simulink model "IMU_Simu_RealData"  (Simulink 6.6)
settings: Solver=ode45  StartTime=0.0  StopTime=33.332  RelTol=1e-3
undefined symbols (not defined in the file or in its folder): float, gaind, polesd, tustin, zerosd

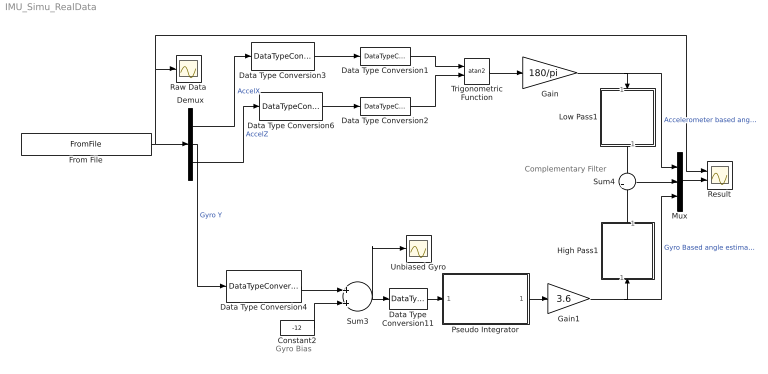
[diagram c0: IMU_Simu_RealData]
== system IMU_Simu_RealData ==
  note: Gyro Bias
  note: Complementary Filter
  Constant2 : Constant  Value=-12  SampleTime=-1
  Data Type Conversion1 : DataTypeConversion  OutDataTypeMode=single  OutScaling="[ (80/(2048*2^4))  0]"
  Data Type Conversion11 : DataTypeConversion  OutDataTypeMode=double  OutScaling="[ (80/(2048*2^4))  0]"
  Data Type Conversion2 : DataTypeConversion  OutDataTypeMode=single  OutScaling="[ (80/(2048*2^4))  0]"
  Data Type Conversion3 : DataTypeConversion  OutDataTypeMode=Specify via dialog  OutDataType=sfix(12)  OutScaling=[1/502.5*1000 0]  ConvertRealWorld=Stored Integer (SI)
  Data Type Conversion4 : DataTypeConversion  OutDataTypeMode=Specify via dialog  OutDataType=sfix(12)  OutScaling="[ (160/4096)  0]"  ConvertRealWorld=Stored Integer (SI)
  Data Type Conversion6 : DataTypeConversion  OutDataTypeMode=Specify via dialog  OutDataType=sfix(12)  OutScaling=[1/486*1000 0]  ConvertRealWorld=Stored Integer (SI)
  Demux : Demux  Outputs=3
  From File : FromFile  FileName=AxelX_GyroY_AxelZ3.mat  SampleTime=.001
  Gain : Gain  Gain=180/pi  OutDataTypeMode=Specify via dialog  OutDataType=float('double')
  Gain1 : Gain  Gain=3.6  OutDataTypeMode=Specify via dialog  OutDataType=float('double')
  High Pass1 : Subsystem  Orientation=up  mask(DiscretizedZeroPole){Zeros=[0], Poles=[-.5], Gain=1, AbsTol=auto, SampleTime=.001, method=tustin, Wc=1}
      mask prompts: Zeros "Zeros (enter in s-main:)"; Poles "Poles (enter in s-domain:)"; Gain "Gain (enter in s-domain:)"; AbsTol "Absolute tolerance:"; SampleTime "Sample time:"; Wc "Critical Frequency (Hz):"
      mask help: Continuous mask uses c2d to transform parameters onto the Discrete Zero-Pole block inside.
      mask init:
      | st=SampleTime;
      | if length(st)>1
      |     st=SampleTime(1);
      | end
      | if(st>0)
      |     [zerosd,polesd,gaind] = sldiscutil('disczpk', {st,method,Wc,Zeros,Poles,Gain});
      | end	
      | s = get_param(gcb,'maskvalues');
      | zeross = s{1};
      | poless = s{2};
      | gainss = s{3};
      | %zerosc = eval(zeross);
      | %polesc = eval(poless);
      | %gainsc = eval(gainss);
      | sldiscutil('initzpkmask', st);
      | if(st==0)
      | set_param([gcb '/Zero Pole'], 'AbsoluteTolerance', AbsTol);
      | end
  Low Pass1 : Subsystem  Orientation=down  mask(DiscretizedZeroPole){Zeros=[], Poles=[-.5], Gain=.5, AbsTol=auto, SampleTime=.001, method=tustin, Wc=1}
      mask prompts: Zeros "Zeros (enter in s-main:)"; Poles "Poles (enter in s-domain:)"; Gain "Gain (enter in s-domain:)"; AbsTol "Absolute tolerance:"; SampleTime "Sample time:"; Wc "Critical Frequency (Hz):"
      mask help: Continuous mask uses c2d to transform parameters onto the Discrete Zero-Pole block inside.
      mask init:
      | st=SampleTime;
      | if length(st)>1
      |     st=SampleTime(1);
      | end
      | if(st>0)
      |     [zerosd,polesd,gaind] = sldiscutil('disczpk', {st,method,Wc,Zeros,Poles,Gain});
      | end	
      | s = get_param(gcb,'maskvalues');
      | zeross = s{1};
      | poless = s{2};
      | gainss = s{3};
      | %zerosc = eval(zeross);
      | %polesc = eval(poless);
      | %gainsc = eval(gainss);
      | sldiscutil('initzpkmask', st);
      | if(st==0)
      | set_param([gcb '/Zero Pole'], 'AbsoluteTolerance', AbsTol);
      | end
  Mux : Mux  Inputs=3
  Pseudo Integrator : Subsystem  mask(DiscretizedZeroPole){Zeros=[0 -314], Poles=[-.03 -.03], Gain=(1/314), AbsTol=auto, SampleTime=.001, method=tustin, Wc=1}
      mask prompts: Zeros "Zeros (enter in s-main:)"; Poles "Poles (enter in s-domain:)"; Gain "Gain (enter in s-domain:)"; AbsTol "Absolute tolerance:"; SampleTime "Sample time:"; Wc "Critical Frequency (Hz):"
      mask help: Continuous mask uses c2d to transform parameters onto the Discrete Zero-Pole block inside.
      mask init:
      | st=SampleTime;
      | if length(st)>1
      |     st=SampleTime(1);
      | end
      | if(st>0)
      |     [zerosd,polesd,gaind] = sldiscutil('disczpk', {st,method,Wc,Zeros,Poles,Gain});
      | end	
      | s = get_param(gcb,'maskvalues');
      | zeross = s{1};
      | poless = s{2};
      | gainss = s{3};
      | %zerosc = eval(zeross);
      | %polesc = eval(poless);
      | %gainsc = eval(gainss);
      | sldiscutil('initzpkmask', st);
      | if(st==0)
      | set_param([gcb '/Zero Pole'], 'AbsoluteTolerance', AbsTol);
      | end
  Raw Data : Scope
  Result : Scope  NumInputPorts=2
  Sum3 : Sum
  Sum4 : Sum
  Trigonometric Function : Trigonometry  Operator=atan2  OutputSignalType=real
  Unbiased Gyro : Scope
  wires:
  Demux/1 -> Data Type Conversion3/1  "AccelX"
  Demux/3 -> Data Type Conversion6/1  "AccelZ"
  Trigonometric Function/1 -> Gain/1
  Constant2/1 -> Sum3/2
  Demux/2 -> Data Type Conversion4/1  "Gyro Y"
  Low Pass1/1(Out1) -> Sum4/1
  High Pass1/1(Out1) -> Sum4/2
  Pseudo Integrator/1(Out1) -> Gain1/1
  Gain1/1 -> High Pass1/1(In1), Mux/3  "Gyro Based angle estimation"
  Gain/1 -> Low Pass1/1(In1), Mux/1  "Accelerometer based angle estimation"
  Sum4/1 -> Mux/2
  Data Type Conversion2/1 -> Trigonometric Function/2
  Data Type Conversion1/1 -> Trigonometric Function/1
  From File/1 -> Demux/1, Raw Data/1, Result/1
  Mux/1 -> Result/2
  Data Type Conversion6/1 -> Data Type Conversion2/1
  Data Type Conversion3/1 -> Data Type Conversion1/1
  Data Type Conversion4/1 -> Sum3/1
  Data Type Conversion11/1 -> Pseudo Integrator/1(In1)
  Sum3/1 -> Data Type Conversion11/1, Unbiased Gyro/1

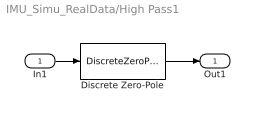
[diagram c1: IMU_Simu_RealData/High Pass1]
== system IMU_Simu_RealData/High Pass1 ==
  In1 : Inport
  Discrete Zero-Pole : DiscreteZeroPole  Zeros=zerosd  Poles=polesd  Gain=gaind  SampleTime=SampleTime
  Out1 : Outport
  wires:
  Discrete Zero-Pole/1 -> Out1/1
  In1/1 -> Discrete Zero-Pole/1

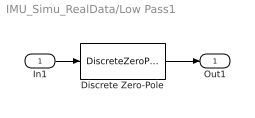
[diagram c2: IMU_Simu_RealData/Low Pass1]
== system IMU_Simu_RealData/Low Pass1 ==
  In1 : Inport
  Discrete Zero-Pole : DiscreteZeroPole  Zeros=zerosd  Poles=polesd  Gain=gaind  SampleTime=SampleTime
  Out1 : Outport
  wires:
  In1/1 -> Discrete Zero-Pole/1
  Discrete Zero-Pole/1 -> Out1/1

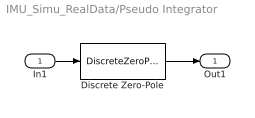
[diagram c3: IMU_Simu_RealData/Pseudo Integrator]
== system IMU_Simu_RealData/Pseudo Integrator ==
  In1 : Inport
  Discrete Zero-Pole : DiscreteZeroPole  Zeros=zerosd  Poles=polesd  Gain=gaind  SampleTime=SampleTime
  Out1 : Outport
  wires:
  Discrete Zero-Pole/1 -> Out1/1
  In1/1 -> Discrete Zero-Pole/1
